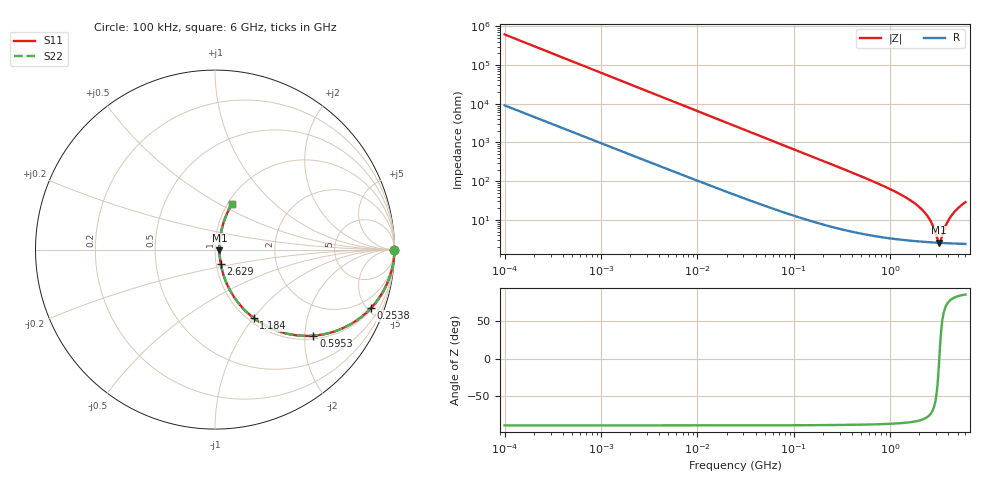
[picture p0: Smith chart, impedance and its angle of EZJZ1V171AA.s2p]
!*** S-Parameter ***
!Copyright  (C)  Panasonic Corporation
!Multilaryer Varistors, Chip Type  Port assignments : Series-thru
!  1  o---GGG---o  2
!Parts No. : EZJZ1V171AA  GND o---------o GND
# HZ  S  RI R  50
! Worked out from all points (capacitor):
!   401 points, 100 kHz to 6 GHz, reference 50 ohm
!   read as one part in series: C = 2.57 pF near 105.7 kHz
!   lowest |Z| = 2.59 ohm at 3.187 GHz (marker M1)
!   series resonance near 3.217 GHz, so ESL is about 950 pH
!   S11 on the Smith chart (normalised r, x): 100 kHz: open; 253.8 MHz: 1.13, -5.28; 595.3 MHz: 1.08, -2.21; 1.184 GHz: 1.06, -1.00; 2.629 GHz: 1.05, -0.17; 6 GHz: 1.05, +0.57
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100000  1 -0.000162  2.41e-06 0.000162  2.41e-06 0.000162  1 -0.000162
631452  1 -0.001  1.6e-05 0.001  1.6e-05 0.001  1 -0.001
3987316  0.9999 -0.0062  0.000134 0.0062  0.000134 0.0062  0.9999 -0.0062
2.44949e7  0.998 -0.0372  0.002 0.0372  0.002 0.0372  0.998 -0.0372
6.777267e7  0.9879 -0.1006  0.0121 0.1006  0.0121 0.1006  0.9879 -0.1006
1.546735e8  0.9452 -0.2173  0.0548 0.2173  0.0548 0.2173  0.9452 -0.2173
2.537656e8  0.8688 -0.3256  0.1312 0.3256  0.1312 0.3256  0.8688 -0.3256
3.833659e8  0.7463 -0.4209  0.2537 0.4209  0.2537 0.4209  0.7463 -0.4209
5.953049e8  0.5483 -0.4797  0.4517 0.4797  0.4517 0.4797  0.5483 -0.4797
9.76689e8  0.2984 -0.432  0.7016 0.432  0.7016 0.432  0.2984 -0.432
1.184061e9  0.2154 -0.3809  0.7846 0.3809  0.7846 0.3809  0.2154 -0.3809
1.558934e9  0.1227 -0.2877  0.8773 0.2877  0.8773 0.2877  0.1227 -0.2877
1.942633e9  0.0717 -0.2035  0.9283 0.2035  0.9283 0.2035  0.0717 -0.2035
2.2912e9  0.0461 -0.1378  0.9539 0.1378  0.9539 0.1378  0.0461 -0.1378
2.628996e9  0.0326 -0.0822  0.9674 0.0822  0.9674 0.0822  0.0326 -0.0822
3.016594e9  0.0258 -0.0262  0.9742 0.0262  0.9742 0.0262  0.0258 -0.0262
3.187187e9  0.0249 -0.00379  0.9751 0.00379  0.9751 0.00379  0.0249 -0.00379
3.367428e9  0.0251 0.0187  0.9749 -0.0187  0.9749 -0.0187  0.0251 0.0187
3.863894e9  0.0301 0.075  0.9699 -0.075  0.9699 -0.075  0.0301 0.075
4.313271e9  0.0391 0.1201  0.9609 -0.1201  0.9609 -0.1201  0.0391 0.1201
5.087202e9  0.0611 0.1874  0.9389 -0.1874  0.9389 -0.1874  0.0611 0.1874
6e9  0.0942 0.2534  0.9058 -0.2534  0.9058 -0.2534  0.0942 0.2534
